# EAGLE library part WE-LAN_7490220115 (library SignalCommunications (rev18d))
WE-LAN LAN Transformer Characteristics Compliant with standards: IEEE 802.3u, IEEE 802.3ab, IEEE 802.3af, IEEE 802.3at and upcoming IEE 802.3bt SMD Applications Ethernet speed up to 10 Gbit/s Power over Ethernet PoE and PoE+ Compliant with most IC’s for Ethernet applications such as Intel, AMD, Microchip and Realtek Hub, Router, Switches, IPcameras, IoT Details see: http://katalog.we-online.de/en/pbs/WE-LAN/7490220115? Created by Yingchun Shan 2016 (C) Wurth Elektronik
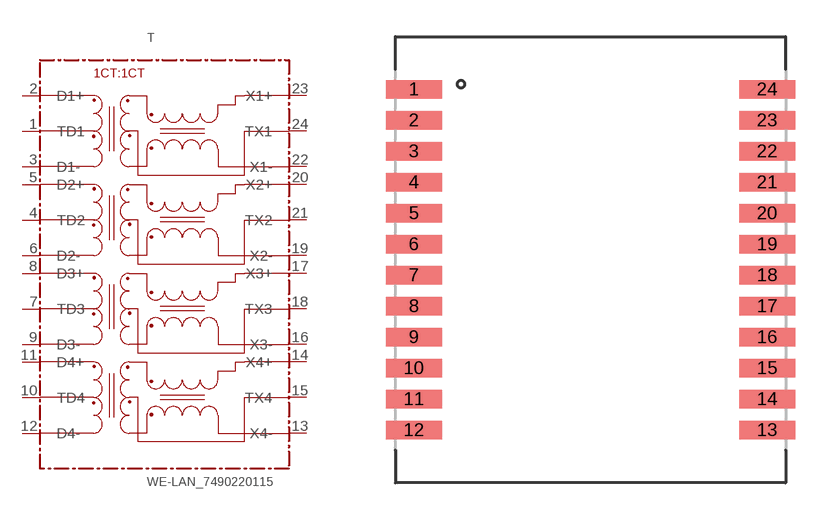
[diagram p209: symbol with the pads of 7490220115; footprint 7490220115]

Designator prefix T

## WE-LAN_7490220115  [7490220115]
1  TD1
2  D1+
3  D1-
4  TD2
5  D2+
6  D2-
7  TD3
8  D3+
9  D3-
10  TD4
11  D4+
12  D4-
13  X4-
14  X4+
15  TX4
16  X3-
17  X3+
18  TX3
19  X2-
20  X2+
21  TX2
22  X1-
23  X1+
24  TX1

## Footprint 7490220115 (pad centres in mm)
smd 2.29 x 0.76: 1 -7.24,6.985; 2 -7.24,5.715; 3 -7.24,4.445; 4 -7.24,3.175; 5 -7.24,1.905; 6 -7.24,0.635; 7 -7.24,-0.635; 8 -7.24,-1.905; 9 -7.24,-3.175; 10 -7.24,-4.445; 11 -7.24,-5.715; 12 -7.24,-6.985; 13 7.24,-6.985; 14 7.24,-5.715; 15 7.24,-4.445; 16 7.24,-3.175; 17 7.24,-1.905; 18 7.24,-0.635; 19 7.24,0.635; 20 7.24,1.905; 21 7.24,3.175; 22 7.24,4.445; 23 7.24,5.715; 24 7.24,6.985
